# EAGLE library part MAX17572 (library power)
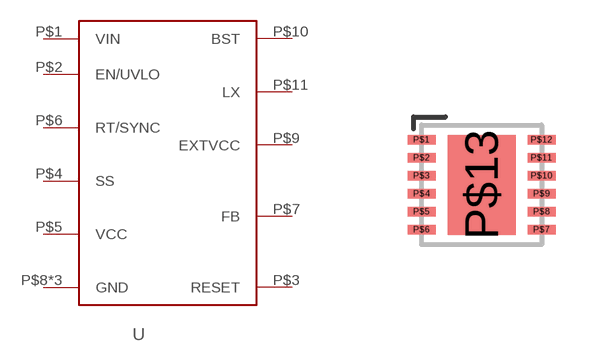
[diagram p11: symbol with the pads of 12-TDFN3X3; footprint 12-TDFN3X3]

Designator prefix U

## MAX17572  [12-TDFN3X3]
P$1  VIN
P$2  EN/UVLO
P$3  RESET
P$4  SS
P$5  VCC
P$6  RT/SYNC
P$7  FB
P$8  GND
P$9  EXTVCC
P$10  BST
P$11  LX
P$12  GND
P$13  GND

## Footprint 12-TDFN3X3 (pad centres in mm)
smd 0.7 x 0.23: P$1 -1.5,1.125; P$2 -1.5,0.675; P$3 -1.5,0.225; P$4 -1.5,-0.225; P$5 -1.5,-0.675; P$6 -1.5,-1.125; P$7 1.5,-1.125; P$8 1.5,-0.675; P$9 1.5,-0.225; P$10 1.5,0.225; P$11 1.5,0.675; P$12 1.5,1.125
smd 1.7 x 2.5: P$13 0,0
